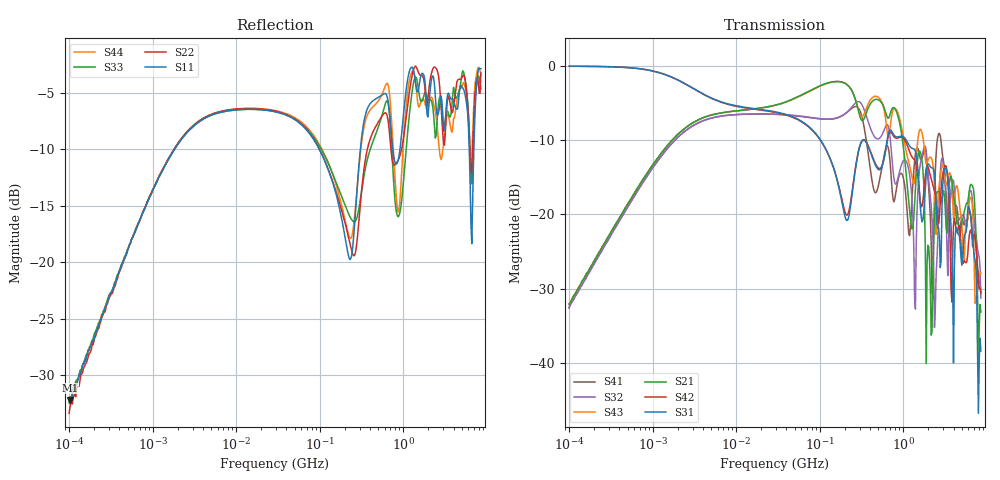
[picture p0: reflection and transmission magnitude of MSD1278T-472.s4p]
# MHz S MA R 50
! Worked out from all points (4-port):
!   498 points, 100 kHz to 8.5 GHz, reference 50 ohm
!   strongest paths, dB at 100 kHz, 1.698 MHz, 29.49 MHz, 500.7 MHz, 8.5 GHz:
!     S31: -0.1, -1.5, -6.2, -13.9, -38.4
!     S42: -0.1, -1.5, -6.3, -13.8, -30.7
!     S21: -32.1, -10.0, -5.3, -4.6, -33.1
!     S43: -32.0, -10.1, -5.3, -4.2, -27.9
!     S32: -32.5, -10.5, -6.5, -9.8, -31.3
!     S41: -32.6, -10.5, -6.5, -16.3, -30.5
!   lowest |S11| = -32.2 dB at 102.3 kHz (marker M1), VSWR 1.05, Z = 50.1 + j2.46 ohm
!   |S11| at or under -10 dB: 98.9 MHz to 306.6 MHz (207.7 MHz wide, 102 % of centre); 747.1 MHz to 914.1 MHz (167 MHz wide, 20.1 % of centre); 6.168 GHz to 7.006 GHz (838.5 MHz wide, 12.7 % of centre)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
0.1  0.02494 83.8  0.02474 86.0  0.9929 -1.4  0.02332 -94.7
     0.02474 86.0  0.02146 88.3  0.02374 -94.6  0.9934 -1.4
     0.9929 -1.4  0.02374 -94.6  0.0239 87.2  0.02504 85.0
     0.02332 -94.7  0.9934 -1.4  0.02504 85.0  0.02481 90.7
0.1023101  0.02456 85.8  0.0252 86.1  0.9934 -1.5  0.0243 -94.4
           0.0252 86.1  0.02274 87.1  0.02425 -94.3  0.9934 -1.4
           0.9934 -1.5  0.02425 -94.3  0.0254 88.0  0.02539 85.4
           0.0243 -94.4  0.9934 -1.4  0.02539 85.4  0.02382 90.4
3.368415  0.4102 29.9  0.4272 32.7  0.6837 -21.1  0.4081 -151.1
          0.4272 32.7  0.4138 30.1  0.4087 -151.2  0.6812 -21.4
          0.6837 -21.1  0.4087 -151.2  0.4099 30.0  0.4275 32.8
          0.4081 -151.1  0.6812 -21.4  0.4275 32.8  0.4138 30.2
163.5102  0.1884 -79.1  0.784 -27.4  0.1652 -84.4  0.4469 64.8
          0.784 -27.4  0.1949 -75.2  0.4461 66.6  0.1675 -83.5
          0.1652 -84.4  0.4461 66.6  0.2168 -79.1  0.7836 -24.8
          0.4469 64.8  0.1675 -83.5  0.7836 -24.8  0.209 -82.6
2260.241  0.6665 167.6  0.03835 -102.4  0.2047 128.2  0.02673 -55.3
          0.03835 -102.4  0.716 175.1  0.07045 69.5  0.1571 109.6
          0.2047 128.2  0.07045 69.5  0.4835 172.4  0.218 85.8
          0.02673 -55.3  0.1571 109.6  0.218 85.8  0.5209 166.6
2713.323  0.4844 117.5  0.1413 124.9  0.06935 32.6  0.3499 114.0
          0.1413 124.9  0.6105 95.1  0.1457 153.1  0.09739 -110.8
          0.06935 32.6  0.1457 153.1  0.534 135.8  0.1631 84.1
          0.3499 114.0  0.09739 -110.8  0.1631 84.1  0.31 108.4
8500  0.717 -50.7  0.02201 -116.4  0.012 -75.5  0.03 -148.2
      0.02201 -116.4  0.6859 -40.0  0.02724 129.2  0.02924 -110.4
      0.012 -75.5  0.02724 129.2  0.5842 -43.6  0.04028 -25.2
      0.03 -148.2  0.02924 -110.4  0.04028 -25.2  0.6725 -50.1
